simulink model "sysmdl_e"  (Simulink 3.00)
settings: Solver=ode45  SolverMode=SingleTasking  StartTime=0.0  StopTime=10.0  RelTol=1e-3  AbsTol=1e-6
undefined symbols (not defined in the file or in its folder): pow

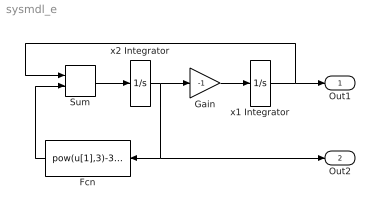
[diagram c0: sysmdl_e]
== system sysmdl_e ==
  Fcn : Fcn  Orientation=left  Expr=pow(u[1],3)-3*u[1]
  Gain : Gain  Gain=-1  SaturateOnIntegerOverflow=on
  Sum : Sum  Inputs=++  SaturateOnIntegerOverflow=on
  x1 Integrator : Integrator  ExternalReset=none  InitialConditionSource=internal  InitialCondition=0  LimitOutput=off  UpperSaturationLimit=inf  LowerSaturationLimit=-inf  ShowSaturationPort=off  ShowStatePort=off  AbsoluteTolerance=auto
  x2 Integrator : Integrator  ExternalReset=none  InitialConditionSource=internal  InitialCondition=0  LimitOutput=off  UpperSaturationLimit=inf  LowerSaturationLimit=-inf  ShowSaturationPort=off  ShowStatePort=off  AbsoluteTolerance=auto
  Out1 : Outport  Port=1
  Out2 : Outport  Port=2
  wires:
  x1 Integrator/1 -> Out1/1, Sum/1
  Fcn/1 -> Sum/2
  x2 Integrator/1 -> Out2/1, Fcn/1, Gain/1
  Sum/1 -> x2 Integrator/1
  Gain/1 -> x1 Integrator/1
